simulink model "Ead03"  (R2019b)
settings: Solver=FixedStepDiscrete  StartTime=0.0  StopTime=6  FixedStep=1  RelTol=1e-3

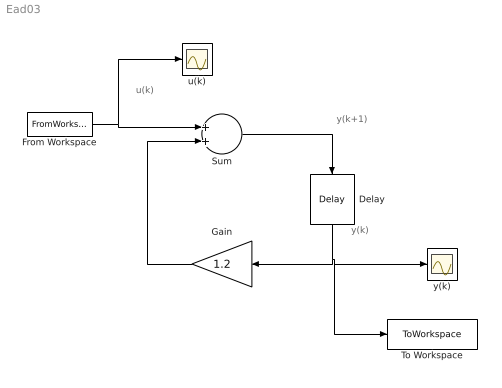
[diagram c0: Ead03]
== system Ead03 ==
  note: y(k+1)
  note: y(k)
  note: u(k)
  Delay : Delay  DelayLength=1  InitialCondition=10
  From Workspace : FromWorkspace  VariableName=u  SampleTime=1
  Gain : Gain  Gain=1.2
  Sum : Sum
  To Workspace : ToWorkspace  VariableName=y  SaveFormat=Timeseries  SampleTime=-1
  u(k) : Scope
  y(k) : Scope
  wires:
  Delay/1 -> To Workspace/1, y(k)/1, Gain/1
  Gain/1 -> Sum/2
  Sum/1 -> Delay/1
  From Workspace/1 -> u(k)/1, Sum/1
